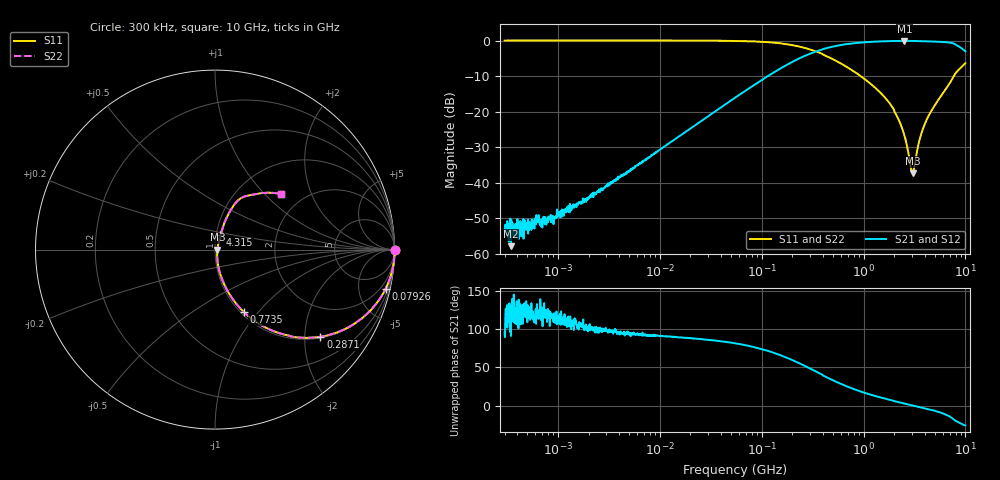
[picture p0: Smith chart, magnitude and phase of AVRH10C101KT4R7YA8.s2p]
! S-Parameter Data Generated by TDK Corporation
! Copyright(C) 2023 TDK Corporation.
! All Rights Reserved.
! TDK P/N: AVRH10C101KT4R7YA8 (Varistor)
! Property: V1mA=115V
! Size(LxWxT): 1x0.5x0.5mm
! Model Type: s2p (Touchstone File Format Version 1.0)
! Frequency: DC=Yes Start=0.3MHz Stop=10000MHz 1602points Log-sweep
! Model Generated on Oct. 12, 2023
! Port Assignments:
!  1 ---N--- 2
! Applicable Conditions:
!  Temperature = 25 degC
!  DC Bias Voltage = 0 V
!  Small Signal Operation
! Terms and conditions regarding TDK Simulation Models
! (1)This simulation model is being provided solely for informational purposes. Please refer to the specifications of the products in terms of detailed characteristics of such products.
! (2)In no event shall TDK Corporation of any of its subsidiaries be liable for any loss or damage arising, directly or indirectly,
!  From any information contained in this simulation model, including, but not limited to loss or damages arising from any inaccuracies, omissions or errors in connection with such information.
! (3)Any and all copyrights on this simulation model are owned by TDK Corporation.
!  Duplication or redistribution of this simulation model without prior written permission from TDK Corporation is prohibited.
! (4)This simulation model is subject to any modification or change without any prior notice.
! (5)Neither TDK Corporation nor any of its subsidiaries shall make any warranty, express or implied,
!  Including but not limited to the correctness, implied warranties of merchantability and fitness for a particular purpose with respect to this simulation models.
! (6)The use of this simulation model shall be deemed to have consented to the terms and conditions hereof.
# Hz S MA R 50
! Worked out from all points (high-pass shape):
!   1601 points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, 300 kHz to 10 GHz, reference 50 ohm
!   highest |S21| = -0.10 dB at 2.523 GHz (marker M1); lowest = -57.9 dB at 346 kHz (marker M2)
!   |S21| within 3 dB of the highest: 340.7 MHz to end of sweep
!   lowest |S11| = -37.3 dB at 3.032 GHz (marker M3), VSWR 1.03, Z = 51.4 - j0.105 ohm
!   |S11| at or under -10 dB: 935.8 MHz to 7.69 GHz (6.755 GHz wide, 157 % of centre)
!   |S22| runs from -37.3 to 0.0 dB; largest |S21 - S12| = 0
!   S11 on the Smith chart (normalised r, x): 300 kHz: open; 79.26 MHz: 0.98, -8.71; 287.1 MHz: 1.03, -2.39; 773.5 MHz: 1.03, -0.84; 4.315 GHz: 1.05, +0.17; 10 GHz: 1.55, +1.24
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300000  1 -0.1  0.002196 95.4  0.002196 95.4  1 -0.1
346000  1 -0.1  0.001277 91.0  0.001277 91.0  1 -0.1
394300  1.001 -0.1  0.001745 136.5  0.001745 136.5  1.001 -0.1
918536  1.002 -0.2  0.003086 120.8  0.003086 120.8  1.002 -0.2
1702530  1.001 -0.3  0.005378 102.7  0.005378 102.7  1.001 -0.3
9678460  1.001 -1.6  0.02814 91.4  0.02814 91.4  1.001 -1.6
5.47723e7  0.9887 -9.0  0.1568 81.4  0.1568 81.4  0.9887 -9.0
7.92618e7  0.9753 -12.9  0.2239 77.2  0.2239 77.2  0.9753 -12.9
1.55331e8  0.9103 -24.2  0.4102 65.5  0.4102 65.5  0.9103 -24.2
2.87054e8  0.7618 -39.6  0.6376 49.6  0.6376 49.6  0.7618 -39.6
3.12869e8  0.7328 -42.0  0.6696 47.1  0.6696 47.1  0.7328 -42.0
7.73471e8  0.381 -65.3  0.9095 22.4  0.9095 22.4  0.381 -65.3
1.76763e9  0.1361 -78.0  0.9808 7.8  0.9808 7.8  0.1361 -78.0
2.1898e9  0.07948 -78.7  0.9874 4.5  0.9874 4.5  0.07948 -78.7
2.52335e9  0.04589 -74.4  0.9887 2.6  0.9887 2.6  0.04589 -74.4
2.90615e9  0.01676 -40.6  0.9873 0.6  0.9873 0.6  0.01676 -40.6
3.03211e9  0.01361 -4.3  0.9864 0.1  0.9864 0.1  0.01361 -4.3
3.15807e9  0.01691 29.8  0.9854 -0.5  0.9854 -0.5  0.01691 29.8
3.76687e9  0.05335 65.3  0.9789 -2.8  0.9789 -2.8  0.05335 65.3
4.31469e9  0.08483 69.1  0.973 -4.7  0.973 -4.7  0.08483 69.1
7.06105e9  0.2545 67.6  0.9332 -14.6  0.9332 -14.6  0.2545 67.6
1e10  0.4796 40.2  0.7055 -26.0  0.7055 -26.0  0.4796 40.2
